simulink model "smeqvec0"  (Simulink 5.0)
settings: Solver=ode45  StartTime=0.0  StopTime=5  MaxStep=1e-3  RelTol=1e-4  AbsTol=1e-4
InitFcn:
  | smdef0vec
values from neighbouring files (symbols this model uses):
  Bm = 0.10    (= 0.1)    [IMabc2.m]    (also in imabcparam.m = 0.01; IMabcrun0.m = 0.01; IMabcrun1.m = 0.001; IMcur0.m = 1e-06)
  H = 0.60    (= 0.6)    [IMabc2.m]    (also in IMcur0.m = 0.3; imdef0vec.m = 0.3; imdef1vec.m = 0.3; imdef2vec.m = 0.3)
  n0 = 0.98    [imdef0vec.m]    (also in imdef1vec.m = 0.978; imdef2vec.m; imdefrotflux.m; imdefSIvec1.m = 0.95)
  Ra = .95    (= 0.95)    [altwdgs.m]    (also in Ccurverun.m = 0.018)
  Te0 = 0.75/wo*p*(Is*conj(Is)*Req)    [imdefSIvec1.m]
  V = [Vas 0 0].'    [Actac.m]    (also in acttrcalc1.m = str2num(get(h,'string')); im3d.m = eval(get(hVs,'String')); IMabc2.m = [vas vbs vcs 0 0 0]'; IMabcf0.m = [vas vbs vcs 0 0 0]')
  wo = 2*pi*freq0    [calc0.m]    (also in IMabc2.m = 376.991118431; imabcparam.m = 376.991118431; IMabcrun0.m = 376.991118431; IMabcrun1.m = 376.991118431)
undefined symbols (not defined in the file or in its folder): delta0, fa0, fk0, L_1, phif0, Rf, Rkd, Rkq, vf0
libraries: simulink x1

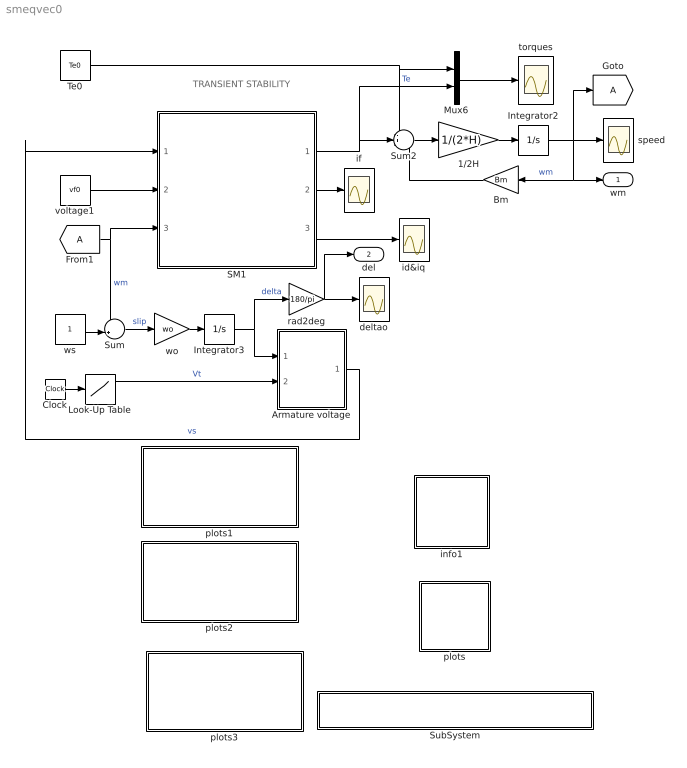
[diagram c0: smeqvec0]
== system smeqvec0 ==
  note: TRANSIENT STABILITY
  1/2H : Gain  Gain=1/(2*H)
  Armature voltage : Subsystem
  Bm : Gain  Orientation=left  Gain=Bm
  Clock : Clock
  Integrator2 : Integrator  InitialCondition=n0
  Integrator3 : Integrator  InitialCondition=delta0
  Look-Up Table : Lookup  InputValues=[0 0.1 0.1 0.2 0.2 3]  OutputValues=[V V 0 0 V V]
  Mux6 : Mux  Inputs=2
  SM1 : Subsystem
  SubSystem : Subsystem
  Sum : Sum  Inputs=-+|
  Sum2 : Sum  Inputs=-+-
  Te0 : Constant  Value=Te0
  deltao : Scope
  id&iq : Scope
  if : Scope
  info1 : Subsystem
  plots : Subsystem
  plots1 : Subsystem
  plots2 : Subsystem
  plots3 : Subsystem
  rad2deg : Gain  Gain=180/pi
  speed : Scope
  torques : Scope
  voltage1 : Constant  Value=vf0
  wo : Gain  Gain=wo
  ws : Constant
  wm : Outport
  del : Outport  Port=2
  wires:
  Mux6/1 -> torques/1
  voltage1/1 -> SM1/2(vf)
  SM1/2(if) -> if/1
  Sum2/1 -> 1/2H/1
  1/2H/1 -> Integrator2/1
  SM1/1(Te) -> Sum2/2, Mux6/2  "Te"
  Bm/1 -> Sum2/3
  Integrator2/1 -> speed/1, [A], Bm/1, wm/1  "wm"
  Te0/1 -> Mux6/1, Sum2/1
  ws/1 -> Sum/2
  Sum/1 -> wo/1  "slip"
  wo/1 -> Integrator3/1
  Armature voltage/1(vs) -> SM1/1(vs)  "vs"
  Integrator3/1 -> Armature voltage/1(delta), rad2deg/1  "delta"
  SM1/3(ia) -> id&iq/1
  rad2deg/1 -> deltao/1, del/1
  Clock/1 -> Look-Up Table/1
  Look-Up Table/1 -> Armature voltage/2(Vt)  "Vt"
  [A] -> SM1/3(wm), Sum/1  "wm"

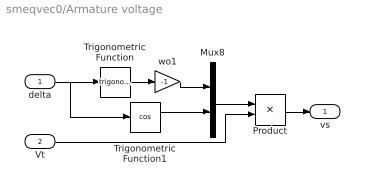
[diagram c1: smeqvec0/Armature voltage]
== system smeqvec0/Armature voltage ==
  delta : Inport
  Vt : Inport  Port=2
  Mux8 : Mux  Inputs=2
  Product : Product
  Trigonometric Function : Trigonometry
  Trigonometric Function1 : Trigonometry  Operator=cos
  wo1 : Gain  Gain=-1
  vs : Outport
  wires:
  delta/1 -> Trigonometric Function/1, Trigonometric Function1/1
  Trigonometric Function/1 -> wo1/1
  Mux8/1 -> Product/1
  wo1/1 -> Mux8/1
  Trigonometric Function1/1 -> Mux8/2
  Product/1 -> vs/1
  Vt/1 -> Product/2

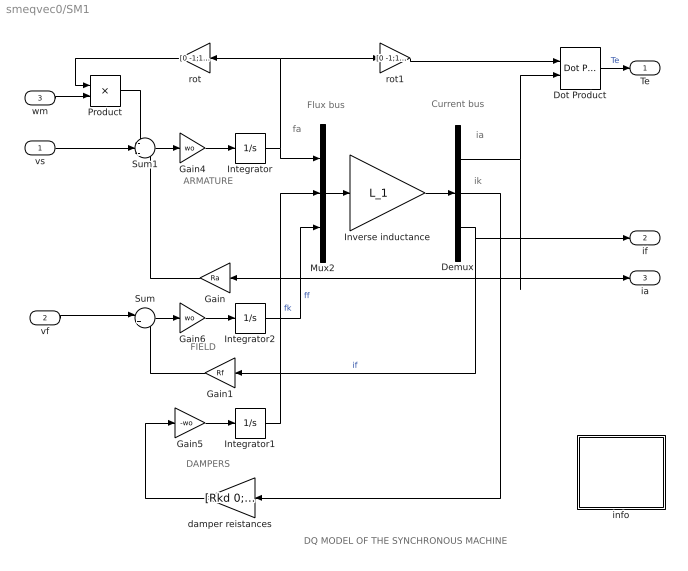
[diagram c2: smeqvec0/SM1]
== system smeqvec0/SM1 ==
  note: DAMPERS
  note: ARMATURE
  note: fa
  note: ia
  note: FIELD
  note: DQ MODEL OF THE SYNCHRONOUS MACHINE
  note: Flux bus
  note: Current bus
  note: ik
  vs : Inport
  vf : Inport  Port=2
  wm : Inport  Port=3
  Demux : Demux  Outputs=3
  Dot Product : simulink/Math Operations/Dot Product
  Gain : Gain  Orientation=left  Gain=Ra
  Gain1 : Gain  Orientation=left  Gain=Rf
  Gain4 : Gain  Gain=wo
  Gain5 : Gain  Gain=-wo
  Gain6 : Gain  Gain=wo
  Integrator : Integrator  InitialCondition=fa0
  Integrator1 : Integrator  InitialCondition=fk0
  Integrator2 : Integrator  InitialCondition=phif0
  Inverse inductance : Gain  Gain=L_1  Multiplication=Matrix(K*u)
  Mux2 : Mux  Inputs=3
  Product : Product
  Sum : Sum  Inputs=|+-
  Sum1 : Sum  Inputs=-+-
  damper reistances : Gain  Orientation=left  Gain=[Rkd 0;0 Rkq]  Multiplication=Matrix(K*u)
  info : Subsystem
  rot : Gain  Orientation=left  Gain=[0 -1;1 0]  Multiplication=Matrix(K*u)
  rot1 : Gain  Gain=[0 -1;1 0]  Multiplication=Matrix(K*u)
  Te : Outport
  if : Outport  Port=2
  ia : Outport  Port=3
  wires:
  Product/1 -> Sum1/1
  rot/1 -> Product/1
  wm/1 -> Product/2
  Gain5/1 -> Integrator1/1
  damper reistances/1 -> Gain5/1
  Integrator/1 -> Mux2/1, rot/1, rot1/1
  Sum1/1 -> Gain4/1
  Gain4/1 -> Integrator/1
  vs/1 -> Sum1/2
  Gain/1 -> Sum1/3
  Gain6/1 -> Integrator2/1
  Sum/1 -> Gain6/1
  vf/1 -> Sum/1
  Gain1/1 -> Sum/2
  rot1/1 -> Dot Product/1
  Demux/1 -> Gain/1, ia/1, Dot Product/2
  Dot Product/1 -> Te/1  "Te"
  Mux2/1 -> Inverse inductance/1
  Inverse inductance/1 -> Demux/1
  Integrator1/1 -> Mux2/2  "fk"
  Integrator2/1 -> Mux2/3  "ff"
  Demux/2 -> damper reistances/1
  Demux/3 -> if/1, Gain1/1  "if"

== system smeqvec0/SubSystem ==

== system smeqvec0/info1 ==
  note: Synchronous machine transients
  note: This demonstration illustrates the dynamics of a synchronous machine following the sudden application and removal of a three-phase short circuit at the terminals. To modify the parameters and loading conditions, click the yellow block. Start the simulation. Four models of the synchronous machine are provided: 1) A complete model (5th-order) 2) Armature transients ignored by setting dfa/dt=0 (3rd-order) 3) Both armature transients and damper effects are neglected (1st-order) 4) Constant field flux linkage (zero-order)

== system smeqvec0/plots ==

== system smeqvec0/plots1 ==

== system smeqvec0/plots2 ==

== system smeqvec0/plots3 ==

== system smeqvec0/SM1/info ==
  note: This demonstration illustrates the dynamics of a synchronous generator, initially at no load, following a three-phase short circuit at the terminals.
  note: Synchronous machine transients under shortcircuit
